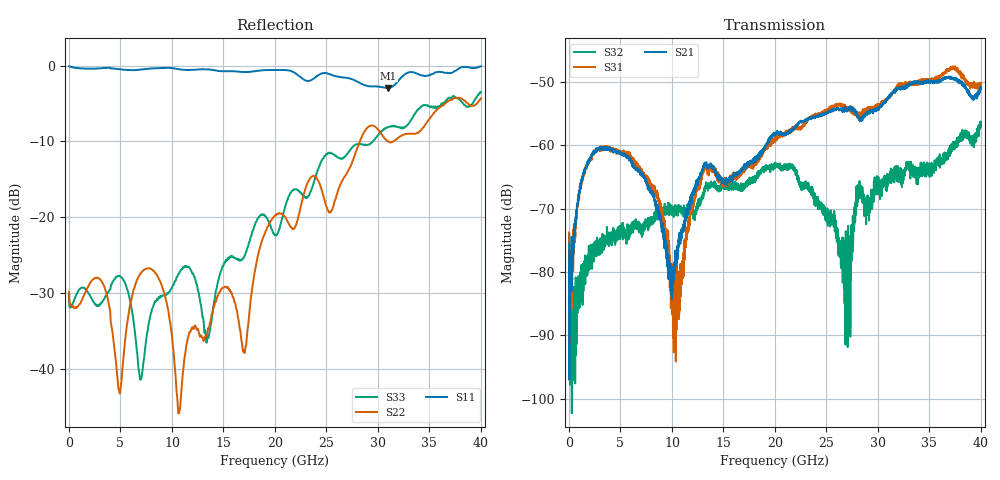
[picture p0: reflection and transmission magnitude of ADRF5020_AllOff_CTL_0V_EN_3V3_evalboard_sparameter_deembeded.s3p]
! Device:  ADRF5020
! Description: SOI MMIC SPDT Non-Reflective Switch
! Frequency:  0.1 -  30 GHz
! Ports:
! 	RFC	= Port 1
!	RF1	= Port 2
!	RF2	= Port 3
! Vdd:  +3.3 Volt
! Vss:  -2.5 Volt
! Control:  0/+3.3 Volt
! State:  All Off (Vctl= 0 V, Ven= 3.3 V)
! Data:	Data was collected using a calibrated network analyzer with AFR software.
!	Fixtures were calculated using AFR and fixturing was applied to collect
!	this Deembedded  S Parameter data of ADRF5020.
! Note:	Analog Devices supplies this data as a sample of measured data at the package pin
!	for this product.  Your particular data for this product may vary.
!	Data was taken at 25 degrees C.
!	Analog Devices reserves the right to change this data at anytime.
# Hz S  dB  R 50
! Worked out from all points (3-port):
!   4000 points, 10 MHz to 40 GHz, reference 50 ohm
!   strongest paths, dB at 10 MHz, 10.01 GHz, 20.01 GHz, 30.01 GHz, 40 GHz:
!     S21: -75.6, -81.9, -58.5, -54.1, -50.8
!     S31: -73.8, -81.1, -59.1, -53.8, -50.4
!     S32: -84.6, -70.2, -63.5, -66.7, -56.8
!   lowest |S11| = -3.0 dB at 31 GHz (marker M1), VSWR 5.92, Z = 77.5 - j123 ohm
!   |S11| at or under -10 dB: nowhere
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1e7  -0.08 -0.4  -75.51 -24.8  -82.75 -97.5
     -75.65 13.1  -29.77 148.4  -88.39 168.6
     -73.76 -72.5  -84.62 19.1  -30.17 146.3
2.75e9  -0.39 -33.5  -60.71 40.8  -60.80 41.6
        -60.81 42.2  -27.93 160.4  -75.52 69.9
        -60.78 40.6  -77.02 81.5  -31.57 168.2
4.91e9  -0.47 -54.3  -61.05 24.6  -61.18 23.3
        -61.04 24.3  -43.13 161.1  -73.80 73.4
        -61.29 21.8  -74.02 71.5  -27.70 -152.7
6.94e9  -0.54 -79.6  -64.44 10.4  -63.88 0.5
        -64.46 11.1  -27.37 155.1  -72.82 81.3
        -64.18 4.0  -73.36 78.6  -41.28 -138.8
9.16e9  -0.31 -103.5  -73.36 13.6  -71.41 -10.7
        -74.23 8.2  -29.59 -126.5  -71.10 82.1
        -72.21 -4.5  -70.36 82.9  -30.29 -143.3
1.069e10  -0.49 -116.7  -74.56 120.3  -79.30 99.7
          -75.52 124.6  -45.63 22.9  -70.54 79.8
          -80.72 99.4  -70.36 75.7  -27.40 -119.9
2.001e10  -0.60 146.6  -57.95 123.2  -59.14 113.5
          -58.53 123.2  -19.77 -29.4  -63.06 -21.4
          -59.09 115.7  -63.46 -17.8  -22.32 -42.8
2.519e10  -1.08 71.2  -54.79 100.2  -54.29 94.9
          -54.68 101.7  -19.17 -33.9  -70.89 -77.7
          -54.45 93.1  -72.44 -78.1  -11.52 -66.0
3.1e10  -2.96 -33.4  -52.47 61.5  -52.79 56.8
        -52.53 62.9  -10.00 -65.7  -64.60 -73.7
        -52.60 55.9  -65.82 -69.0  -8.10 -92.8
4e10  -0.10 -137.6  -50.82 8.4  -50.22 -8.8
      -50.77 7.5  -4.32 -117.6  -57.29 115.7
      -50.36 -7.0  -56.82 118.6  -3.50 -137.6
